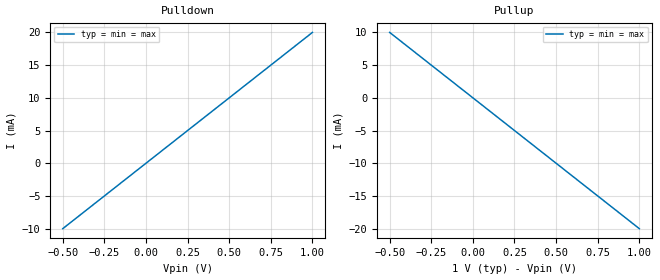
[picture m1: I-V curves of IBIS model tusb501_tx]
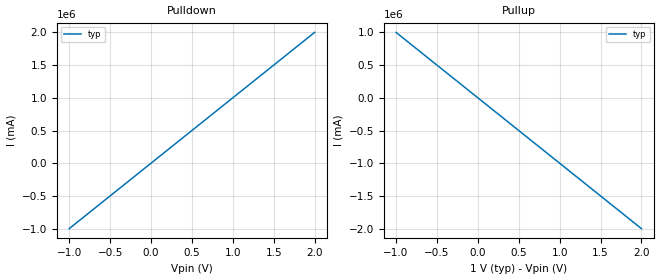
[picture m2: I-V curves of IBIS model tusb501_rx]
[IBIS Ver]   5.0
[File Name]  tusb501.ibs
[File Rev]   1.0
[Component]  tusb501
[Manufacturer] Texas Instruments Incorporated
[Package]
R_pkg  0.0   NA   NA
L_pkg  0.0   NA   NA
C_pkg  0.0   NA   NA
[Pin]   signal_name   model_name   R_pin L_pin  C_pin
1p   Tx_p   tusb501_tx
1n   Tx_n   tusb501_tx
2p   Rx_p   tusb501_rx
2n   Rx_n   tusb501_rx
[Diff_Pin] inv_pin vdiff tdelay_typ tdelay_min tdelay_max
2p   2n   NA   NA   NA   NA
1p   1n   NA   NA   NA   NA
| Models and submodels in the file (2): tusb501_tx (Output), tusb501_rx (Input)
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[Model] tusb501_tx
Model_type Output
C_comp 0p 0p 0p
Cref = 0
Vref = 0.5
Rref = 50
Vmeas = 0.5
[Temperature_Range] 25 125 0
[Voltage Range] 1 1 1
[Algorithmic Model]
Executable Windows_VisualC++ExpressEdition9.0.30729_32 tusb501_tx.dll tusb501_tx.ami
[End Algorithmic Model]
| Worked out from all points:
|   slope of the pulldown table from 0 to 0.15 V, typ, clamps not added: 50 ohm
|   slope of the pullup table from 0 to 0.15 V, typ, clamps not added: 50 ohm
[Pulldown]
-500mV    -10mA      -10mA      -10mA
0V        0A         0A         0A
1V        20mA       20mA       20mA
[Pullup]
-500mV    10mA       10mA       10mA
0V        0A         0A         0A
1V        -20mA      -20mA      -20mA
[GND Clamp]
-500mV    0A         0A         0A
0V        0A         0A         0A
1V        0A         0A         0A
[Power Clamp]
-500mV    0A         0A         0A
0V        0A         0A         0A
1V        0A         0A         0A
[Ramp]
dV/dt_r 0.45/1p 0.45/1p 0.45/1p
dV/dt_f 0.45/1p 0.45/1p 0.45/1p
R_load=0.001Ohms
[Model] tusb501_rx
Model_type Input
C_comp 0p 0p 0p
Vinl = 0.3
Vinh = 0.7
[Temperature_Range] 25 125 0
[Voltage Range] 1.0 1.0 1.0
[Algorithmic Model]
Executable Windows_VisualC++ExpressEdition9.0.30729_32 tusb501_rx.dll tusb501_rx.ami
[End Algorithmic Model]
[Ramp]
|   typ   min   max
dV/dt_r   0.8/1.0ps   NA   NA
dV/dt_f   0.8/1.0ps   NA   NA
R_load = 0.001ohm
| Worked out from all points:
|   slope of the pulldown table from 0 to 0.15 V, typ, clamps not added: 1 mohm
|   slope of the pullup table from 0 to 0.15 V, typ, clamps not added: 1 mohm
[Pulldown]
|Voltage I(typ)   I(min)   I(max)
-1V       -1kA       NA         NA
0V        0A         NA         NA
2V        2kA        NA         NA
[Pullup]
-1V       1kA        NA         NA
0V        0A         NA         NA
2V        -2kA       NA         NA
[GND Clamp]
-1V       0A         0A         0A
0V        0A         0A         0A
2V        0A         0A         0A
[Power Clamp]
-1V       0A         0A         0A
0V        0A         0A         0A
2V        0A         0A         0A
